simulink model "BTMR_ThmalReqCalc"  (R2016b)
settings: Solver=FixedStepDiscrete  StartTime=0.0  StopTime=10.0  FixedStep=0.1  RelTol=1e-3  EnableMultiTasking=on
undefined symbols (not defined in the file or in its folder): BMS_cntThmStbNum_C, BTMR_cntThmalReqVal_C, BTMR_flgCoolPwrCal_C, BTMR_pChrgClntPwrLv1_C, BTMR_pChrgClntPwrLv2_C, BTMR_pChrgClntPwrLv3_C, BTMR_pChrgClntPwrLv4_C, BTMR_pChrgClntPwrLv5_C, BTMR_pChrgClntPwrLv6_C, BTMR_pCoolPwrVal_C, BTMR_pHtgACPwrReq_C, BTMR_pHtgDCPwrReq_C, BTMR_pHtgDrvPwrReq_C, BTMR_pHtgsStage1_CUR, BTMR_pHtgsStage2_CUR, BTMR_pNormClntPwrLv1_C, BTMR_pNormClntPwrLv2_C, BTMR_pNormClntPwrLv3_C, BTMR_r861BrsDrvSoc_C, BTMR_r861HtgDrvSoc_C, BTMR_r891BrsDrvSoc_C, BTMR_r891HtgDrvSoc_C, BTMR_rCoolClbFlg_C, BTMR_rFlashClbFlg_C, BTMR_rHeatClbFlg_C, BTMR_t861BrsDiffLv0Temp_C, BTMR_t861BrsDiffLv1Temp_C, BTMR_t861CoolChrgAces2Temp_C, BTMR_t861CoolChrgAces3Temp_C, BTMR_t861CoolChrgAcesTemp_C, BTMR_t861CoolChrgDiffDebTemp_C, BTMR_t861CoolChrgEndDiffTemp_C, BTMR_t861CoolChrgExitLv2Temp_C, BTMR_t861CoolChrgExitLv3Temp_C, BTMR_t861CoolChrgExitTemp_C, BTMR_t861CoolChrgIntLv0Temp_C, BTMR_t861CoolChrgIntLv1Temp_C, BTMR_t861CoolChrgIntLv2Temp_C, BTMR_t861CoolChrgIntLv3Temp_C, BTMR_t861CoolChrgIntLv4Temp_C, BTMR_t861CoolChrgIntLv5Temp_C, BTMR_t861CoolDCDebTemp_C, BTMR_t861CoolNormAcesTemp_C, BTMR_t861CoolNormDiffDebTemp_C, BTMR_t861CoolNormEndDiffTemp_C, BTMR_t861CoolNormExitLv2Temp_C, BTMR_t861CoolNormExitLv3Temp_C, BTMR_t861CoolNormExitTemp_C, BTMR_t861CoolNormIntLv0Temp_C, BTMR_t861CoolNormIntLv1Temp_C, BTMR_t861CoolNormLv2Temp_C, BTMR_t861CoolNormLv3Temp_C, BTMR_t861HtgACDiffDebTemp_C, BTMR_t861HtgACEndDiffTemp_C, BTMR_t861HtgACStartHiTemp_C, BTMR_t861HtgACStartLoTemp_C, BTMR_t861HtgACStopTemp_C, BTMR_t861HtgDCDiffDebTemp_C, BTMR_t861HtgDCEndDiffTemp_C, BTMR_t861HtgDCIntLv0Temp_C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
libraries: AIWAYS_Powertrain_BMS_lib x78, simulink x9
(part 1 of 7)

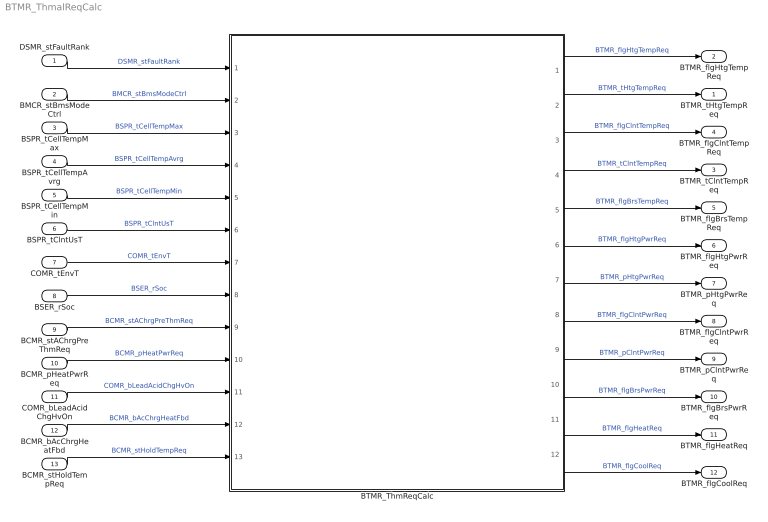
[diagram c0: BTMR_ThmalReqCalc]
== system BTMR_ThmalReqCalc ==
  DSMR_stFaultRank : Inport
  BMCR_stBmsModeCtrl : Inport  Port=2
  BSPR_tCellTempMax : Inport  Port=3
  BSPR_tCellTempAvrg : Inport  Port=4
  BSPR_tCellTempMin : Inport  Port=5
  BSPR_tClntUsT : Inport  Port=6
  COMR_tEnvT : Inport  Port=7
  BSER_rSoc : Inport  Port=8
  BCMR_stAChrgPreThmReq : Inport  Port=9
  BCMR_pHeatPwrReq : Inport  Port=10
  COMR_bLeadAcidChgHvOn : Inport  Port=11
  BCMR_bAcChrgHeatFbd : Inport  Port=12
  BCMR_stHoldTempReq : Inport  Port=13
  BTMR_ThmReqCalc : Subsystem
  BTMR_tHtgTempReq : Outport
  BTMR_flgHtgTempReq : Outport  Port=2
  BTMR_tClntTempReq : Outport  Port=3
  BTMR_flgClntTempReq : Outport  Port=4
  BTMR_flgBrsTempReq : Outport  Port=5
  BTMR_flgHtgPwrReq : Outport  Port=6
  BTMR_pHtgPwrReq : Outport  Port=7
  BTMR_flgClntPwrReq : Outport  Port=8
  BTMR_pClntPwrReq : Outport  Port=9
  BTMR_flgBrsPwrReq : Outport  Port=10
  BTMR_flgHeatReq : Outport  Port=11
  BTMR_flgCoolReq : Outport  Port=12
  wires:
  BMCR_stBmsModeCtrl/1 -> BTMR_ThmReqCalc/2(BMCR_stBmsModeCtrl)  "BMCR_stBmsModeCtrl"
  DSMR_stFaultRank/1 -> BTMR_ThmReqCalc/1(DSMR_stFaultRank)  "DSMR_stFaultRank"
  BSPR_tCellTempMax/1 -> BTMR_ThmReqCalc/3(BSPR_tCellTempMax)  "BSPR_tCellTempMax"
  BSPR_tCellTempAvrg/1 -> BTMR_ThmReqCalc/4(BSPR_tCellTempAvrg)  "BSPR_tCellTempAvrg"
  BSPR_tCellTempMin/1 -> BTMR_ThmReqCalc/5(BSPR_tCellTempMin)  "BSPR_tCellTempMin"
  BTMR_ThmReqCalc/2(BTMR_tHtgTempReq) -> BTMR_tHtgTempReq/1  "BTMR_tHtgTempReq"
  COMR_tEnvT/1 -> BTMR_ThmReqCalc/7(COMR_tEnvT)  "COMR_tEnvT"
  BSPR_tClntUsT/1 -> BTMR_ThmReqCalc/6(BSPR_tClntUsT)  "BSPR_tClntUsT"
  BSER_rSoc/1 -> BTMR_ThmReqCalc/8(BSER_rSoc)  "BSER_rSoc"
  BCMR_pHeatPwrReq/1 -> BTMR_ThmReqCalc/10(BCMR_pHeatPwrReq)  "BCMR_pHeatPwrReq"
  BCMR_stAChrgPreThmReq/1 -> BTMR_ThmReqCalc/9(BCMR_stAChrgPreThmReq)  "BCMR_stAChrgPreThmReq"
  BTMR_ThmReqCalc/1(BTMR_flgHtgTempReq) -> BTMR_flgHtgTempReq/1  "BTMR_flgHtgTempReq"
  BTMR_ThmReqCalc/5(BTMR_flgBrsTempReq) -> BTMR_flgBrsTempReq/1  "BTMR_flgBrsTempReq"
  BTMR_ThmReqCalc/4(BTMR_tClntTempReq) -> BTMR_tClntTempReq/1  "BTMR_tClntTempReq"
  BTMR_ThmReqCalc/3(BTMR_flgClntTempReq) -> BTMR_flgClntTempReq/1  "BTMR_flgClntTempReq"
  COMR_bLeadAcidChgHvOn/1 -> BTMR_ThmReqCalc/11(COMR_bLeadAcidChgHvOn)  "COMR_bLeadAcidChgHvOn"
  BCMR_bAcChrgHeatFbd/1 -> BTMR_ThmReqCalc/12(BCMR_bAcChrgHeatFbd)  "BCMR_bAcChrgHeatFbd"
  BTMR_ThmReqCalc/6(BTMR_flgHtgPwrReq) -> BTMR_flgHtgPwrReq/1  "BTMR_flgHtgPwrReq"
  BTMR_ThmReqCalc/7(BTMR_pHtgPwrReq) -> BTMR_pHtgPwrReq/1  "BTMR_pHtgPwrReq"
  BTMR_ThmReqCalc/8(BTMR_flgClntPwrReq) -> BTMR_flgClntPwrReq/1  "BTMR_flgClntPwrReq"
  BTMR_ThmReqCalc/9(BTMR_pClntPwrReq) -> BTMR_pClntPwrReq/1  "BTMR_pClntPwrReq"
  BTMR_ThmReqCalc/10(BTMR_flgBrsPwrReq) -> BTMR_flgBrsPwrReq/1  "BTMR_flgBrsPwrReq"
  BCMR_stHoldTempReq/1 -> BTMR_ThmReqCalc/13(BCMR_stHoldTempReq)  "BCMR_stHoldTempReq"
  BTMR_ThmReqCalc/11(BTMR_flgHeatReq) -> BTMR_flgHeatReq/1  "BTMR_flgHeatReq"
  BTMR_ThmReqCalc/12(BTMR_flgCoolReq) -> BTMR_flgCoolReq/1  "BTMR_flgCoolReq"

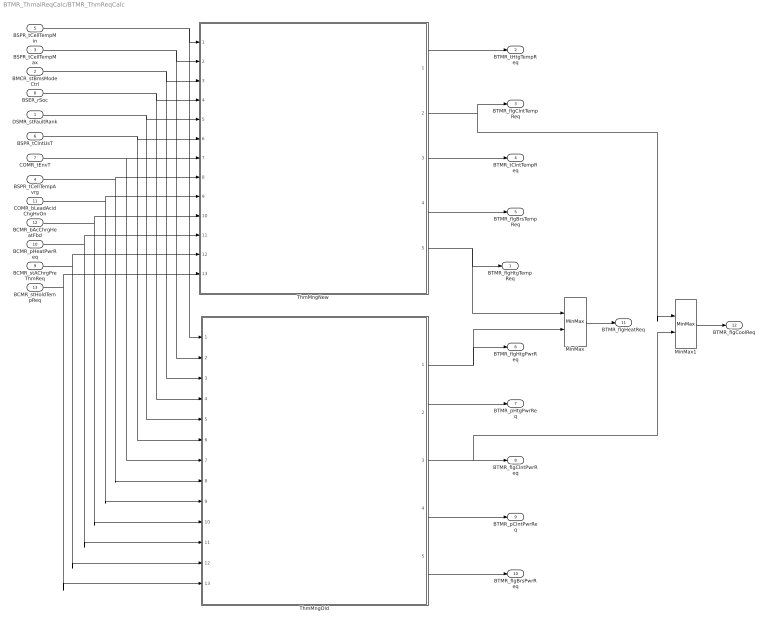
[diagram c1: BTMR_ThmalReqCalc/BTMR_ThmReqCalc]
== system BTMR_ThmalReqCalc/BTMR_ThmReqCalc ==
  DSMR_stFaultRank : Inport
  BMCR_stBmsModeCtrl : Inport  Port=2
  BSPR_tCellTempMax : Inport  Port=3
  BSPR_tCellTempAvrg : Inport  Port=4
  BSPR_tCellTempMin : Inport  Port=5
  BSPR_tClntUsT : Inport  Port=6
  COMR_tEnvT : Inport  Port=7
  BSER_rSoc : Inport  Port=8
  BCMR_stAChrgPreThmReq : Inport  Port=9
  BCMR_pHeatPwrReq : Inport  Port=10
  COMR_bLeadAcidChgHvOn : Inport  Port=11
  BCMR_bAcChrgHeatFbd : Inport  Port=12
  BCMR_stHoldTempReq : Inport  Port=13
  MinMax : MinMax  Function=max  Inputs=2
  MinMax1 : MinMax  Function=max  Inputs=2
  ThmMngNew : Subsystem
  ThmMngOld : Subsystem
  BTMR_flgHtgTempReq : Outport
  BTMR_tHtgTempReq : Outport  Port=2
  BTMR_flgClntTempReq : Outport  Port=3
  BTMR_tClntTempReq : Outport  Port=4
  BTMR_flgBrsTempReq : Outport  Port=5
  BTMR_flgHtgPwrReq : Outport  Port=6
  BTMR_pHtgPwrReq : Outport  Port=7
  BTMR_flgClntPwrReq : Outport  Port=8
  BTMR_pClntPwrReq : Outport  Port=9
  BTMR_flgBrsPwrReq : Outport  Port=10
  BTMR_flgHeatReq : Outport  Port=11
  BTMR_flgCoolReq : Outport  Port=12
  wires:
  BSPR_tCellTempMin/1 -> ThmMngOld/1(BSPR_tCellTempMin), ThmMngNew/1(BSPR_tCellTempMin)
  BSPR_tCellTempMax/1 -> ThmMngOld/2(BSPR_tCellTempMax), ThmMngNew/2(BSPR_tCellTempMax)
  BMCR_stBmsModeCtrl/1 -> ThmMngOld/3(BMCR_stBmsModeCtrl), ThmMngNew/3(BMCR_stBmsModeCtrl)
  BSER_rSoc/1 -> ThmMngOld/4(BSER_rSoc), ThmMngNew/4(BSER_rSoc)
  DSMR_stFaultRank/1 -> ThmMngOld/5(DSMR_stFaultRank), ThmMngNew/5(DSMR_stFaultRank)
  BSPR_tClntUsT/1 -> ThmMngOld/6(BSPR_tClntUsT), ThmMngNew/6(BSPR_tClntUsT)
  COMR_tEnvT/1 -> ThmMngOld/7(COMR_tEnvT), ThmMngNew/7(COMR_tEnvT)
  BSPR_tCellTempAvrg/1 -> ThmMngOld/8(BSPR_tCellTempAvrg), ThmMngNew/8(BSPR_tCellTempAvrg)
  COMR_bLeadAcidChgHvOn/1 -> ThmMngOld/9(COMR_bLeadAcidChgHvOn), ThmMngNew/9(COMR_bLeadAcidChgHvOn)
  BCMR_bAcChrgHeatFbd/1 -> ThmMngOld/10(BCMR_bAcChrgHeatFbd), ThmMngNew/10(BCMR_bAcChrgHeatFbd)
  BCMR_pHeatPwrReq/1 -> ThmMngOld/11(BCMR_pHeatPwrReq), ThmMngNew/11(BCMR_pHeatPwrReq)
  BCMR_stAChrgPreThmReq/1 -> ThmMngOld/12(BCMR_stAChrgPreThmReq), ThmMngNew/12(BCMR_stAChrgPreThmReq)
  ThmMngNew/5(BTMR_flgHtgTempReq_891) -> MinMax/1, BTMR_flgHtgTempReq/1
  ThmMngNew/1(BTMR_tHtgTempReq_891) -> BTMR_tHtgTempReq/1
  ThmMngNew/2(BTMR_flgClntTempReq_891) -> MinMax1/1, BTMR_flgClntTempReq/1
  ThmMngNew/3(BTMR_tClntTempReq_891) -> BTMR_tClntTempReq/1
  ThmMngNew/4(BTMR_flgBrsTempReq_891) -> BTMR_flgBrsTempReq/1
  ThmMngOld/1(BTMR_flgHtgPwrReq_861) -> BTMR_flgHtgPwrReq/1, MinMax/2
  ThmMngOld/2(BTMR_pHtgPwrReq_861) -> BTMR_pHtgPwrReq/1
  ThmMngOld/3(BTMR_flgClntPwrReq_861) -> MinMax1/2, BTMR_flgClntPwrReq/1
  ThmMngOld/4(BTMR_pClntPwrReq_861) -> BTMR_pClntPwrReq/1
  ThmMngOld/5(BTMR_flgBrsPwrReq_861) -> BTMR_flgBrsPwrReq/1
  BCMR_stHoldTempReq/1 -> ThmMngNew/13(BCMR_stHoldTempReq), ThmMngOld/13(BCMR_stHoldTempReq)
  MinMax/1 -> BTMR_flgHeatReq/1
  MinMax1/1 -> BTMR_flgCoolReq/1

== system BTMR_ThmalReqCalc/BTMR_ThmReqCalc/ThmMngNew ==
  BSPR_tCellTempMin : Inport
  BSPR_tCellTempMax : Inport  Port=2
  BMCR_stBmsModeCtrl : Inport  Port=3
  BSER_rSoc : Inport  Port=4
  DSMR_stFaultRank : Inport  Port=5
  BSPR_tClntUsT : Inport  Port=6
  COMR_tEnvT : Inport  Port=7
  BSPR_tCellTempAvrg : Inport  Port=8
  COMR_bLeadAcidChgHvOn : Inport  Port=9
  BCMR_bAcChrgHeatFbd : Inport  Port=10
  BCMR_pHeatPwrReq : Inport  Port=11
  BCMR_stAChrgPreThmReq : Inport  Port=12
  BCMR_stHoldTempReq : Inport  Port=13
  BTMR_ThmFlgTempCalc : Subsystem
  BTMR_ThmLogSgnsCalc : Subsystem
  BTMR_ThmSgnsPros : Subsystem
  BTMR_ThmStsCalc : Subsystem
  BTMR_tHtgTempReq_891 : Outport
  BTMR_flgClntTempReq_891 : Outport  Port=2
  BTMR_tClntTempReq_891 : Outport  Port=3
  BTMR_flgBrsTempReq_891 : Outport  Port=4
  BTMR_flgHtgTempReq_891 : Outport  Port=5
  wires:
  COMR_tEnvT/1 -> BTMR_ThmSgnsPros/7(COMR_tEnvT)
  BTMR_ThmStsCalc/1(stBrsSts) -> BTMR_ThmFlgTempCalc/1(stBrsSts)
  BTMR_ThmStsCalc/2(stHtgSts) -> BTMR_ThmFlgTempCalc/2(stHtgSts)
  BTMR_ThmStsCalc/3(stCoolSts) -> BTMR_ThmFlgTempCalc/3(stCoolSts)
  BTMR_ThmFlgTempCalc/5(BTMR_flgBrsTempReq) -> BTMR_flgBrsTempReq_891/1
  BTMR_ThmFlgTempCalc/1(BTMR_flgHtgTempReq) -> BTMR_flgHtgTempReq_891/1
  BTMR_ThmFlgTempCalc/2(BTMR_tHtgTempReq) -> BTMR_tHtgTempReq_891/1
  BTMR_ThmFlgTempCalc/3(BTMR_flgClntTempReq) -> BTMR_flgClntTempReq_891/1
  BTMR_ThmFlgTempCalc/4(BTMR_tClntTempReq) -> BTMR_tClntTempReq_891/1
  BSPR_tCellTempMin/1 -> BTMR_ThmSgnsPros/1(BSPR_tCellTempMin)
  BSPR_tCellTempMax/1 -> BTMR_ThmSgnsPros/2(BSPR_tCellTempMax)
  BSER_rSoc/1 -> BTMR_ThmSgnsPros/4(BSER_rSoc)
  BMCR_stBmsModeCtrl/1 -> BTMR_ThmSgnsPros/3(BMCR_stBmsModeCtrl)
  DSMR_stFaultRank/1 -> BTMR_ThmSgnsPros/5(DSMR_stFaultRank)
  BSPR_tClntUsT/1 -> BTMR_ThmSgnsPros/6(BSPR_tClntUsT)
  BTMR_ThmSgnsPros/3(BTMR_flgThmEnaTempSgns) -> BTMR_ThmLogSgnsCalc/3(BTMR_flgThmEnaTempSgns)
  BTMR_ThmSgnsPros/4(BTMR_flgBrsTempSgns) -> BTMR_ThmStsCalc/4(BTMR_flgBrsTempSgns), BTMR_ThmLogSgnsCalc/4(BTMR_flgBrsTempSgns)
  BTMR_ThmSgnsPros/1(BTMR_flgBMSStsSgns) -> BTMR_ThmLogSgnsCalc/1(BTMR_flgBMSStsSgns)
  BTMR_ThmSgnsPros/2(BTMR_flgSOCSgns) -> BTMR_ThmLogSgnsCalc/2(BTMR_flgSOCSgns)
  BTMR_ThmSgnsPros/6(BTMR_flgCoolTempSgns) -> BTMR_ThmLogSgnsCalc/6(BTMR_flgCoolTempSgns), BTMR_ThmFlgTempCalc/4(BTMR_flgCoolTempSgns)
  BTMR_ThmSgnsPros/5(BTMR_flgHtgTempSgns) -> BTMR_ThmLogSgnsCalc/5(BTMR_flgHtgTempSgns)
  BTMR_ThmLogSgnsCalc/1(BTMR_flgBTMREnaSgns) -> BTMR_ThmStsCalc/1(BTMR_flgBTMREnaSgns)
  BTMR_ThmLogSgnsCalc/2(BTMR_flgBTMRDnaSgns) -> BTMR_ThmStsCalc/2(BTMR_flgBTMRDnaSgns)
  BTMR_ThmSgnsPros/7(BTMR_flgThmEndSgns) -> BTMR_ThmStsCalc/3(BTMR_flgThmEndSgns)
  BSPR_tCellTempAvrg/1 -> BTMR_ThmSgnsPros/8(BSPR_tCellTempAvrg)
  COMR_bLeadAcidChgHvOn/1 -> BTMR_ThmSgnsPros/9(COMR_bLeadAcidChgHvOn)
  BCMR_pHeatPwrReq/1 -> BTMR_ThmFlgTempCalc/5(BCMR_pHeatPwrReq)
  BCMR_stAChrgPreThmReq/1 -> BTMR_ThmFlgTempCalc/6(BCMR_stAChrgPreThmReq)
  BCMR_bAcChrgHeatFbd/1 -> BTMR_ThmSgnsPros/10(BCMR_bAcChrgHeatFbd)
  BCMR_stHoldTempReq/1 -> BTMR_ThmFlgTempCalc/7(BCMR_stHoldTempReq)

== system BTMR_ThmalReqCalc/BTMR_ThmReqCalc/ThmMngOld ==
  BSPR_tCellTempMin : Inport
  BSPR_tCellTempMax : Inport  Port=2
  BMCR_stBmsModeCtrl : Inport  Port=3
  BSER_rSoc : Inport  Port=4
  DSMR_stFaultRank : Inport  Port=5
  BSPR_tClntUsT : Inport  Port=6
  COMR_tEnvT : Inport  Port=7
  BSPR_tCellTempAvrg : Inport  Port=8
  COMR_bLeadAcidChgHvOn : Inport  Port=9
  BCMR_bAcChrgHeatFbd : Inport  Port=10
  BCMR_pHeatPwrReq : Inport  Port=11
  BCMR_stAChrgPreThmReq : Inport  Port=12
  BCMR_stHoldTempReq : Inport  Port=13
  BTMR_ThmFlgPwrCalc : Subsystem
  BTMR_ThmInSgnsPros : Subsystem
  BTMR_ThmLogSgnsCalc : Subsystem
  BTMR_ThmStsCalc : Subsystem
  BTMR_flgHtgPwrReq_861 : Outport
  BTMR_pHtgPwrReq_861 : Outport  Port=2
  BTMR_flgClntPwrReq_861 : Outport  Port=3
  BTMR_pClntPwrReq_861 : Outport  Port=4
  BTMR_flgBrsPwrReq_861 : Outport  Port=5
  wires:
  COMR_tEnvT/1 -> BTMR_ThmInSgnsPros/7(COMR_tEnvT)
  BTMR_ThmStsCalc/1(stBrsSts) -> BTMR_ThmFlgPwrCalc/1(stBrsSts)
  BTMR_ThmStsCalc/2(stHtgSts) -> BTMR_ThmFlgPwrCalc/2(stHtgSts)
  BTMR_ThmStsCalc/3(stCoolSts) -> BTMR_ThmFlgPwrCalc/3(stCoolSts)
  BTMR_ThmFlgPwrCalc/5(BTMR_flgBrsPwrReq) -> BTMR_flgBrsPwrReq_861/1
  BTMR_ThmFlgPwrCalc/1(BTMR_flgHtgPwrReq) -> BTMR_flgHtgPwrReq_861/1
  BTMR_ThmFlgPwrCalc/2(BTMR_pHtgPwrReq) -> BTMR_pHtgPwrReq_861/1
  BTMR_ThmFlgPwrCalc/3(BTMR_flgClntPwrReq) -> BTMR_flgClntPwrReq_861/1
  BTMR_ThmFlgPwrCalc/4(BTMR_pClntPwrReq) -> BTMR_pClntPwrReq_861/1
  BSPR_tCellTempMin/1 -> BTMR_ThmInSgnsPros/1(BSPR_tCellTempMin)
  BSPR_tCellTempMax/1 -> BTMR_ThmInSgnsPros/2(BSPR_tCellTempMax)
  BSER_rSoc/1 -> BTMR_ThmInSgnsPros/4(BSER_rSoc)
  BMCR_stBmsModeCtrl/1 -> BTMR_ThmInSgnsPros/3(BMCR_stBmsModeCtrl)
  DSMR_stFaultRank/1 -> BTMR_ThmInSgnsPros/5(DSMR_stFaultRank)
  BSPR_tClntUsT/1 -> BTMR_ThmInSgnsPros/6(BSPR_tClntUsT)
  BTMR_ThmInSgnsPros/3(BTMR_flgThmEnaTempSgns) -> BTMR_ThmLogSgnsCalc/3(BTMR_flgThmEnaTempSgns)
  BTMR_ThmInSgnsPros/4(BTMR_flgBrsTempSgns) -> BTMR_ThmLogSgnsCalc/4(BTMR_flgBrsTempSgns), BTMR_ThmStsCalc/4(BTMR_flgBrsTempSgns)
  BTMR_ThmInSgnsPros/1(BTMR_flgBMSStsSgns) -> BTMR_ThmLogSgnsCalc/1(BTMR_flgBMSStsSgns)
  BTMR_ThmInSgnsPros/2(BTMR_flgSOCSgns) -> BTMR_ThmLogSgnsCalc/2(BTMR_flgSOCSgns)
  BTMR_ThmInSgnsPros/6(BTMR_flgCoolTempSgns) -> BTMR_ThmLogSgnsCalc/6(BTMR_flgCoolTempSgns), BTMR_ThmFlgPwrCalc/5(BTMR_flgCoolTempSgns)
  BTMR_ThmInSgnsPros/5(BTMR_flgHtgTempSgns) -> BTMR_ThmLogSgnsCalc/5(BTMR_flgHtgTempSgns), BTMR_ThmFlgPwrCalc/4(BTMR_flgHtgTempSgns)
  BTMR_ThmLogSgnsCalc/1(BTMR_flgBTMREnaSgns) -> BTMR_ThmStsCalc/1(BTMR_flgBTMREnaSgns)
  BTMR_ThmLogSgnsCalc/2(BTMR_flgBTMRDnaSgns) -> BTMR_ThmStsCalc/2(BTMR_flgBTMRDnaSgns)
  BTMR_ThmInSgnsPros/7(BTMR_flgThmEndSgns) -> BTMR_ThmStsCalc/3(BTMR_flgThmEndSgns)
  BTMR_ThmInSgnsPros/8(BTMR_pHtgDCPwrSgns) -> BTMR_ThmFlgPwrCalc/6(BTMR_pHtgDCPwrSgns)
  BSPR_tCellTempAvrg/1 -> BTMR_ThmInSgnsPros/8(BSPR_tCellTempAvrg)
  COMR_bLeadAcidChgHvOn/1 -> BTMR_ThmInSgnsPros/9(COMR_bLeadAcidChgHvOn)
  BCMR_pHeatPwrReq/1 -> BTMR_ThmFlgPwrCalc/7(BCMR_pHeatPwrReq)
  BCMR_stAChrgPreThmReq/1 -> BTMR_ThmFlgPwrCalc/8(BCMR_stAChrgPreThmReq)
  BCMR_bAcChrgHeatFbd/1 -> BTMR_ThmInSgnsPros/10(BCMR_bAcChrgHeatFbd)
  BCMR_stHoldTempReq/1 -> BTMR_ThmFlgPwrCalc/9(BCMR_stHoldTempReq)

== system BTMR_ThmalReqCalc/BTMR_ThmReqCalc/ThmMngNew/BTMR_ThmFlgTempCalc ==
  stBrsSts : Inport
  stHtgSts : Inport  Port=2
  stCoolSts : Inport  Port=3
  BTMR_flgCoolTempSgns : Inport  Port=4
  BCMR_pHeatPwrReq : Inport  Port=5
  BCMR_stAChrgPreThmReq : Inport  Port=6
  BCMR_stHoldTempReq : Inport  Port=7
  BTMR_BrushFlgCalc : Subsystem  TreatAsAtomicUnit=on
  BTMR_CoolFlgTempCalc : Subsystem
  BTMR_HtgFlgTempCalc : Subsystem  TreatAsAtomicUnit=on
  BTMR_flgHtgTempReq : Outport
  BTMR_tHtgTempReq : Outport  Port=2
  BTMR_flgClntTempReq : Outport  Port=3
  BTMR_tClntTempReq : Outport  Port=4
  BTMR_flgBrsTempReq : Outport  Port=5
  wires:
  BTMR_CoolFlgTempCalc/1(BTMR_flgClntTempReq) -> BTMR_flgClntTempReq/1
  BTMR_CoolFlgTempCalc/2(BTMR_tClntTempReq) -> BTMR_tClntTempReq/1
  BTMR_BrushFlgCalc/1(BTMR_flgBrsTempReq) -> BTMR_CoolFlgTempCalc/1(BTMR_flgBrsTempReq), BTMR_flgBrsTempReq/1
  BTMR_HtgFlgTempCalc/1(BTMR_flgHtgTempReq) -> BTMR_flgHtgTempReq/1
  BTMR_HtgFlgTempCalc/2(BTMR_tHtgTempReq) -> BTMR_tHtgTempReq/1
  stBrsSts/1 -> BTMR_BrushFlgCalc/1(stBrsSts)
  stHtgSts/1 -> BTMR_HtgFlgTempCalc/1(stHtgSts)
  stCoolSts/1 -> BTMR_CoolFlgTempCalc/2(stCoolSts)
  BTMR_flgCoolTempSgns/1 -> BTMR_CoolFlgTempCalc/3(BTMR_flgCoolTempSgns)
  BCMR_pHeatPwrReq/1 -> BTMR_HtgFlgTempCalc/2(BCMR_pHeatPwrReq)
  BCMR_stAChrgPreThmReq/1 -> BTMR_HtgFlgTempCalc/3(BCMR_stAChrgPreThmReq)
  BCMR_stHoldTempReq/1 -> BTMR_HtgFlgTempCalc/4(BCMR_stHoldTempReq)

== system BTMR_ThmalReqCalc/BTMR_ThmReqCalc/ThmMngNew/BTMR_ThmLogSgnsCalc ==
  BTMR_flgBMSStsSgns : Inport
  BTMR_flgSOCSgns : Inport  Port=2
  BTMR_flgThmEnaTempSgns : Inport  Port=3
  BTMR_flgBrsTempSgns : Inport  Port=4
  BTMR_flgHtgTempSgns : Inport  Port=5
  BTMR_flgCoolTempSgns : Inport  Port=6
  BTMR_BThmDnaLogCalc : Subsystem
  BTMR_BThmEnaLogCalc : Subsystem
  BTMR_ThmLogPreCalc : Subsystem
  BTMR_flgBTMREnaSgns : Outport
  BTMR_flgBTMRDnaSgns : Outport  Port=2
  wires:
  BTMR_flgBrsTempSgns/1 -> BTMR_BThmDnaLogCalc/2(BTMR_flgBrsTempSgns), BTMR_ThmLogPreCalc/4(BTMR_flgBrsTempSgns)
  BTMR_flgHtgTempSgns/1 -> BTMR_BThmDnaLogCalc/3(BTMR_flgHtgTempSgns)
  BTMR_flgCoolTempSgns/1 -> BTMR_BThmDnaLogCalc/4(BTMR_flgCoolTempSgns)
  BTMR_BThmDnaLogCalc/1(BTMR_flgBThmDnaSgns) -> BTMR_flgBTMRDnaSgns/1
  BTMR_flgBMSStsSgns/1 -> BTMR_ThmLogPreCalc/1(BTMR_flgBMSStsSgns)
  BTMR_flgSOCSgns/1 -> BTMR_BThmEnaLogCalc/4(BTMR_flgSOCSgns), BTMR_BThmDnaLogCalc/1(BTMR_flgSOCSgns), BTMR_ThmLogPreCalc/2(BTMR_flgSOCSgns)
  BTMR_BThmEnaLogCalc/1(BTMR_flgBTMREnaSgns) -> BTMR_flgBTMREnaSgns/1
  BTMR_ThmLogPreCalc/2(BTMR_flgHtgLogSgns) -> BTMR_BThmEnaLogCalc/2(BTMR_flgHtgLogSgns)
  BTMR_ThmLogPreCalc/1(BTMR_flgBrsLogSgns) -> BTMR_BThmEnaLogCalc/1(BTMR_flgBrsLogSgns)
  BTMR_ThmLogPreCalc/3(BTMR_flgCoolLogSgns) -> BTMR_BThmEnaLogCalc/3(BTMR_flgCoolLogSgns)
  BTMR_flgThmEnaTempSgns/1 -> BTMR_ThmLogPreCalc/3(BTMR_flgThmEnaTempSgns)

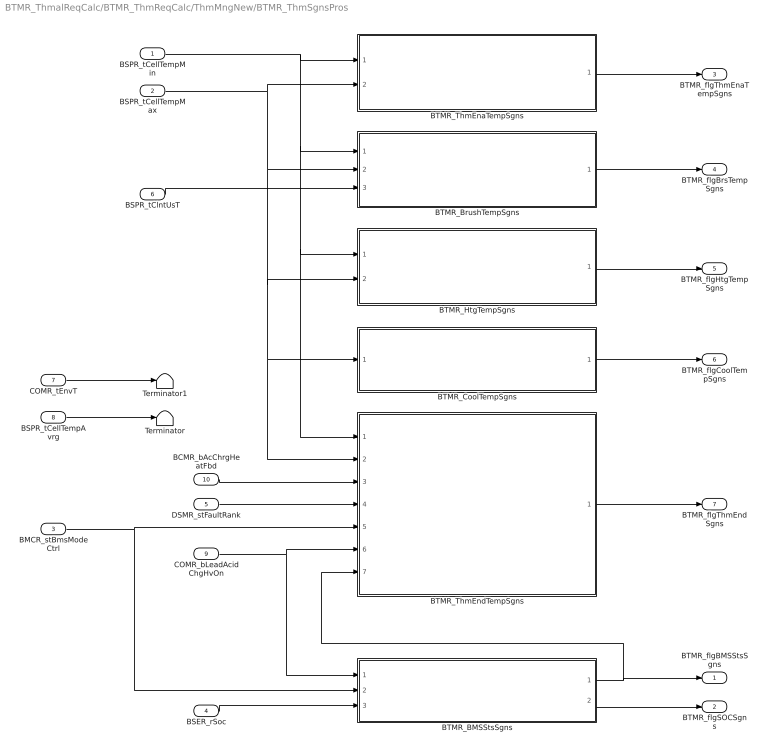
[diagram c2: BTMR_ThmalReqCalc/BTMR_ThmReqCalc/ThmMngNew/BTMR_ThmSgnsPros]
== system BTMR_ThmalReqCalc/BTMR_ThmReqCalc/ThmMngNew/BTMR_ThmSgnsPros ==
  BSPR_tCellTempMin : Inport
  BSPR_tCellTempMax : Inport  Port=2
  BMCR_stBmsModeCtrl : Inport  Port=3
  BSER_rSoc : Inport  Port=4
  DSMR_stFaultRank : Inport  Port=5
  BSPR_tClntUsT : Inport  Port=6
  COMR_tEnvT : Inport  Port=7
  BSPR_tCellTempAvrg : Inport  Port=8
  COMR_bLeadAcidChgHvOn : Inport  Port=9
  BCMR_bAcChrgHeatFbd : Inport  Port=10
  BTMR_BMSStsSgns : Subsystem
  BTMR_BrushTempSgns : Subsystem
  BTMR_CoolTempSgns : Subsystem
  BTMR_HtgTempSgns : Subsystem
  BTMR_ThmEnaTempSgns : Subsystem
  BTMR_ThmEndTempSgns : Subsystem
  Terminator : Terminator
  Terminator1 : Terminator
  BTMR_flgBMSStsSgns : Outport
  BTMR_flgSOCSgns : Outport  Port=2
  BTMR_flgThmEnaTempSgns : Outport  Port=3
  BTMR_flgBrsTempSgns : Outport  Port=4
  BTMR_flgHtgTempSgns : Outport  Port=5
  BTMR_flgCoolTempSgns : Outport  Port=6
  BTMR_flgThmEndSgns : Outport  Port=7
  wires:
  BTMR_ThmEnaTempSgns/1(BTMR_flgThmEnaTempSgns) -> BTMR_flgThmEnaTempSgns/1
  BSPR_tClntUsT/1 -> BTMR_BrushTempSgns/3(BSPR_tClntUsT)
  BTMR_CoolTempSgns/1(BTMR_flgCoolTempSgns) -> BTMR_flgCoolTempSgns/1
  BSER_rSoc/1 -> BTMR_BMSStsSgns/3(BSER_rSoc)
  BTMR_ThmEndTempSgns/1(BTMR_flgThmEndSgns) -> BTMR_flgThmEndSgns/1
  BTMR_BMSStsSgns/1(BTMR_flgBMSSgns) -> BTMR_ThmEndTempSgns/7(BTMR_flgBMSSgns), BTMR_flgBMSStsSgns/1
  BTMR_HtgTempSgns/1(BTMR_flgHtgTempSgns) -> BTMR_flgHtgTempSgns/1
  BTMR_BrushTempSgns/1(BTMR_flgBrsTempSgns) -> BTMR_flgBrsTempSgns/1
  BTMR_BMSStsSgns/2(BTMR_flgSOCSgns) -> BTMR_flgSOCSgns/1
  BMCR_stBmsModeCtrl/1 -> BTMR_BMSStsSgns/2(BMCR_stBmsModeCtrl), BTMR_ThmEndTempSgns/5(BMCR_stBmsModeCtrl)
  DSMR_stFaultRank/1 -> BTMR_ThmEndTempSgns/4(DSMR_stFaultRank)
  BSPR_tCellTempMax/1 -> BTMR_ThmEndTempSgns/2(BSPR_tCellTempMax), BTMR_CoolTempSgns/1(BSPR_tCellTempMax), BTMR_HtgTempSgns/2(BSPR_tCellTempMax), BTMR_BrushTempSgns/2(BSPR_tCellTempMax), BTMR_ThmEnaTempSgns/2(BSPR_tCellTempMax)
  BSPR_tCellTempMin/1 -> BTMR_ThmEndTempSgns/1(BSPR_tCellTempMin), BTMR_HtgTempSgns/1(BSPR_tCellTempMin), BTMR_BrushTempSgns/1(BSPR_tCellTempMin), BTMR_ThmEnaTempSgns/1(BSPR_tCellTempMin)
  BSPR_tCellTempAvrg/1 -> Terminator/1
  COMR_bLeadAcidChgHvOn/1 -> BTMR_BMSStsSgns/1(COMR_bLeadAcidChgHvOn), BTMR_ThmEndTempSgns/6(COMR_bLeadAcidChgHvOn)
  COMR_tEnvT/1 -> Terminator1/1
  BCMR_bAcChrgHeatFbd/1 -> BTMR_ThmEndTempSgns/3(BCMR_bAcChrgHeatFbd)

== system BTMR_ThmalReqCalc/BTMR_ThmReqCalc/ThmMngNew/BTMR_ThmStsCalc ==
  BTMR_flgBTMREnaSgns : Inport
  BTMR_flgBTMRDnaSgns : Inport  Port=2
  BTMR_flgThmEndSgns : Inport  Port=3
  BTMR_flgBrsTempSgns : Inport  Port=4
  BTMR_ThmStsCalc : Stateflow chart  TreatAsAtomicUnit=on
  Bus Selector : BusSelector  OutputSignals=BTMR_flgBrsEna,BTMR_flgHtgDCEna,BTMR_flgHtgACEna,BTMR_flgHtgDrvSEna,BTMR_flgCoolNormEna,BTMR_flgCoolChrgEna
  Bus Selector1 : BusSelector  OutputSignals=BTMR_flgBrsDna,BTMR_flgHtgDCDna,BTMR_flgHtgACDna,BTMR_flgHtgDrvDna,BTMR_flgCoolNormDna,BTMR_flgCoolChrgDna
  Bus Selector2 : BusSelector  OutputSignals=BTMR_flgBrsThmEnd,BTMR_flgHtgDCThmEnd,BTMR_flgHtgACThmEnd,BTMR_flgHtgDrvThmEnd,BTMR_flgCoolNormThmEnd,BTMR_flgCoolChrgThmEnd
  Bus Selector3 : BusSelector  OutputSignals=BTMR_flgBrsInTempSgns
  Bus Selector4 : BusSelector  OutputSignals=BTMR_flgBrsStartTemp
  Data Type Conversion : DataTypeConversion  OutDataTypeStr=uint8
  Data Type Conversion1 : DataTypeConversion  OutDataTypeStr=uint8
  Data Type Conversion2 : DataTypeConversion  OutDataTypeStr=uint8
  stBrsSts : Outport
  stHtgSts : Outport  Port=2
  stCoolSts : Outport  Port=3
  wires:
  BTMR_ThmStsCalc/2(stHtgSts) -> Data Type Conversion1/1
  BTMR_ThmStsCalc/1(stBrsSts) -> Data Type Conversion/1
  BTMR_ThmStsCalc/3(stCoolSts) -> Data Type Conversion2/1
  BTMR_flgBTMREnaSgns/1 -> Bus Selector/1
  Bus Selector/2 -> BTMR_ThmStsCalc/2(HtgDCEna)  "<BTMR_flgHtgDCEna>"
  Bus Selector/1 -> BTMR_ThmStsCalc/1(BrsEna)  "<BTMR_flgBrsEna>"
  Bus Selector/3 -> BTMR_ThmStsCalc/3(HtgACEna)  "<BTMR_flgHtgACEna>"
  Bus Selector/4 -> BTMR_ThmStsCalc/4(HtgDrvEna)  "<BTMR_flgHtgDrvSEna>"
  Bus Selector/5 -> BTMR_ThmStsCalc/5(CoolNormEna)  "<BTMR_flgCoolNormEna>"
  Bus Selector/6 -> BTMR_ThmStsCalc/6(CoolChrgEna)  "<BTMR_flgCoolChrgEna>"
  BTMR_flgBTMRDnaSgns/1 -> Bus Selector1/1
  Bus Selector1/1 -> BTMR_ThmStsCalc/7(BrsDna)  "<BTMR_flgBrsDna>"
  Bus Selector1/2 -> BTMR_ThmStsCalc/8(HtgDCDna)  "<BTMR_flgHtgDCDna>"
  Bus Selector1/3 -> BTMR_ThmStsCalc/9(HtgACDna)  "<BTMR_flgHtgACDna>"
  Bus Selector1/4 -> BTMR_ThmStsCalc/10(HtgDrvDna)  "<BTMR_flgHtgDrvDna>"
  Bus Selector1/5 -> BTMR_ThmStsCalc/11(CoolNormDna)  "<BTMR_flgCoolNormDna>"
  Bus Selector1/6 -> BTMR_ThmStsCalc/12(CoolChrgDna)  "<BTMR_flgCoolChrgDna>"
  BTMR_flgThmEndSgns/1 -> Bus Selector2/1
  Bus Selector2/2 -> BTMR_ThmStsCalc/14(HtgDCThmEnd)  "<BTMR_flgHtgDCThmEnd>"
  Bus Selector2/3 -> BTMR_ThmStsCalc/15(HtgACThmEnd)  "<BTMR_flgHtgACThmEnd>"
  Bus Selector2/4 -> BTMR_ThmStsCalc/16(HtgDrvThmEnd)  "<BTMR_flgHtgDrvThmEnd>"
  Bus Selector2/5 -> BTMR_ThmStsCalc/17(CoolNormThmEnd)  "<BTMR_flgCoolNormThmEnd>"
  Bus Selector2/6 -> BTMR_ThmStsCalc/18(CoolChrgThmEnd)  "<BTMR_flgCoolChrgThmEnd>"
  BTMR_flgBrsTempSgns/1 -> Bus Selector3/1
  Bus Selector3/1 -> Bus Selector4/1  "<BTMR_flgBrsInTempSgns>"
  Bus Selector4/1 -> BTMR_ThmStsCalc/19(BrsStart)  "<BTMR_flgBrsStartTemp>"
  Bus Selector2/1 -> BTMR_ThmStsCalc/13(BrsThmEnd)  "<BTMR_flgBrsThmEnd>"
  Data Type Conversion/1 -> stBrsSts/1
  Data Type Conversion1/1 -> stHtgSts/1
  Data Type Conversion2/1 -> stCoolSts/1

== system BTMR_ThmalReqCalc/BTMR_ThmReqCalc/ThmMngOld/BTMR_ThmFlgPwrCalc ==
  stBrsSts : Inport
  stHtgSts : Inport  Port=2
  stCoolSts : Inport  Port=3
  BTMR_flgHtgTempSgns : Inport  Port=4
  BTMR_flgCoolTempSgns : Inport  Port=5
  BTMR_pHtgDCPwrSgns : Inport  Port=6
  BCMR_pHeatPwrReq : Inport  Port=7
  BCMR_stAChrgPreThmReq : Inport  Port=8
  BCMR_stHoldTempReq : Inport  Port=9
  BTMR_BrushFlgCalc : Subsystem  TreatAsAtomicUnit=on
  BTMR_CoolFlgPwrCalc : Subsystem
  BTMR_HtgFlgPwrCalc : Subsystem  TreatAsAtomicUnit=on
  BTMR_flgHtgPwrReq : Outport
  BTMR_pHtgPwrReq : Outport  Port=2
  BTMR_flgClntPwrReq : Outport  Port=3
  BTMR_pClntPwrReq : Outport  Port=4
  BTMR_flgBrsPwrReq : Outport  Port=5
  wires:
  BTMR_CoolFlgPwrCalc/1(BTMR_flgClntPwrReq) -> BTMR_flgClntPwrReq/1
  BTMR_CoolFlgPwrCalc/2(BTMR_pClntPwrReq) -> BTMR_pClntPwrReq/1
  BTMR_BrushFlgCalc/1(BTMR_flgBrsPwrReq) -> BTMR_CoolFlgPwrCalc/1(BTMR_flgBrsPwrReq), BTMR_flgBrsPwrReq/1
  BTMR_HtgFlgPwrCalc/1(BTMR_flgHtgPwrReq) -> BTMR_flgHtgPwrReq/1
  BTMR_HtgFlgPwrCalc/2(BTMR_pHtgPwrReq) -> BTMR_pHtgPwrReq/1
  stBrsSts/1 -> BTMR_BrushFlgCalc/1(stBrsSts)
  stHtgSts/1 -> BTMR_HtgFlgPwrCalc/1(stHtgSts)
  stCoolSts/1 -> BTMR_CoolFlgPwrCalc/2(stCoolSts)
  BTMR_flgHtgTempSgns/1 -> BTMR_HtgFlgPwrCalc/2(BTMR_flgHtgTempSgns)
  BTMR_pHtgDCPwrSgns/1 -> BTMR_HtgFlgPwrCalc/3(BTMR_pHtgDCPwrSgns)
  BTMR_flgCoolTempSgns/1 -> BTMR_CoolFlgPwrCalc/3(BTMR_flgCoolTempSgns)
  BCMR_pHeatPwrReq/1 -> BTMR_HtgFlgPwrCalc/4(BCMR_pHeatPwrReq)
  BCMR_stAChrgPreThmReq/1 -> BTMR_HtgFlgPwrCalc/5(BCMR_stAChrgPreThmReq)
  BCMR_stHoldTempReq/1 -> BTMR_HtgFlgPwrCalc/6(BCMR_stHoldTempReq)

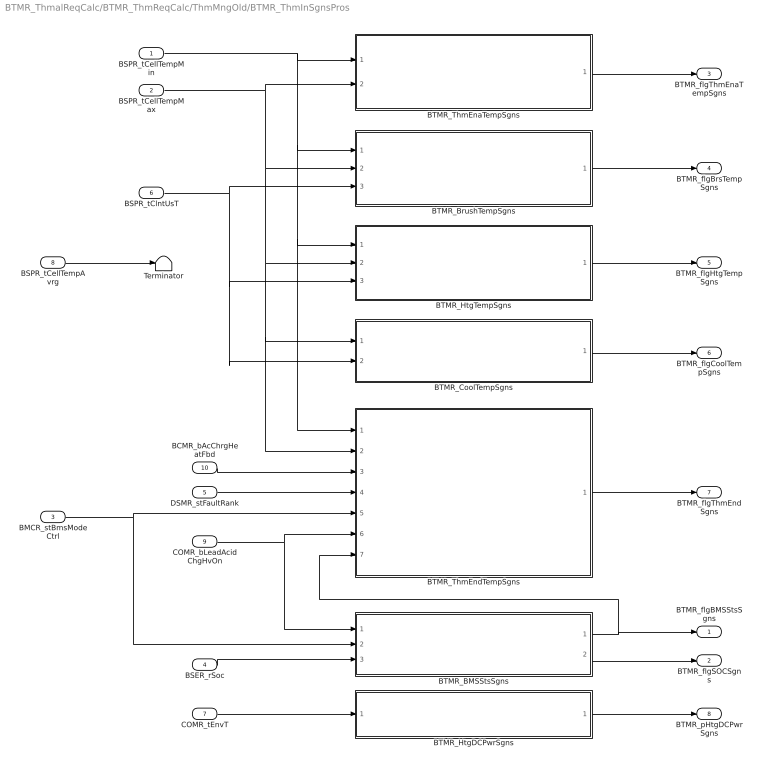
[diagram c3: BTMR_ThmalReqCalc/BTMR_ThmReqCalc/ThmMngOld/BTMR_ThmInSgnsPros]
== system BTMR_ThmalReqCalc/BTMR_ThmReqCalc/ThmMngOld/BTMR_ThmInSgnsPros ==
  BSPR_tCellTempMin : Inport
  BSPR_tCellTempMax : Inport  Port=2
  BMCR_stBmsModeCtrl : Inport  Port=3
  BSER_rSoc : Inport  Port=4
  DSMR_stFaultRank : Inport  Port=5
  BSPR_tClntUsT : Inport  Port=6
  COMR_tEnvT : Inport  Port=7
  BSPR_tCellTempAvrg : Inport  Port=8
  COMR_bLeadAcidChgHvOn : Inport  Port=9
  BCMR_bAcChrgHeatFbd : Inport  Port=10
  BTMR_BMSStsSgns : Subsystem
  BTMR_BrushTempSgns : Subsystem
  BTMR_CoolTempSgns : Subsystem
  BTMR_HtgDCPwrSgns : Subsystem
  BTMR_HtgTempSgns : Subsystem
  BTMR_ThmEnaTempSgns : Subsystem
  BTMR_ThmEndTempSgns : Subsystem
  Terminator : Terminator
  BTMR_flgBMSStsSgns : Outport
  BTMR_flgSOCSgns : Outport  Port=2
  BTMR_flgThmEnaTempSgns : Outport  Port=3
  BTMR_flgBrsTempSgns : Outport  Port=4
  BTMR_flgHtgTempSgns : Outport  Port=5
  BTMR_flgCoolTempSgns : Outport  Port=6
  BTMR_flgThmEndSgns : Outport  Port=7
  BTMR_pHtgDCPwrSgns : Outport  Port=8
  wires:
  BTMR_ThmEnaTempSgns/1(BTMR_flgThmEnaTempSgns) -> BTMR_flgThmEnaTempSgns/1
  BSPR_tClntUsT/1 -> BTMR_CoolTempSgns/2(BSPR_tClntUsT), BTMR_HtgTempSgns/3(BSPR_tClntUsT), BTMR_BrushTempSgns/3(BSPR_tClntUsT)
  BTMR_CoolTempSgns/1(BTMR_flgCoolTempSgns) -> BTMR_flgCoolTempSgns/1
  BSER_rSoc/1 -> BTMR_BMSStsSgns/3(BSER_rSoc)
  BTMR_ThmEndTempSgns/1(BTMR_flgThmEndSgns) -> BTMR_flgThmEndSgns/1
  BTMR_BMSStsSgns/1(BTMR_flgBMSSgns) -> BTMR_ThmEndTempSgns/7(BTMR_flgBMSSgns), BTMR_flgBMSStsSgns/1
  BTMR_HtgTempSgns/1(BTMR_flgHtgTempSgns) -> BTMR_flgHtgTempSgns/1
  BTMR_BrushTempSgns/1(BTMR_flgBrsTempSgns) -> BTMR_flgBrsTempSgns/1
  BTMR_BMSStsSgns/2(BTMR_flgSOCSgns) -> BTMR_flgSOCSgns/1
  BMCR_stBmsModeCtrl/1 -> BTMR_BMSStsSgns/2(BMCR_stBmsModeCtrl), BTMR_ThmEndTempSgns/5(BMCR_stBmsModeCtrl)
  DSMR_stFaultRank/1 -> BTMR_ThmEndTempSgns/4(DSMR_stFaultRank)
  BSPR_tCellTempMax/1 -> BTMR_ThmEndTempSgns/2(BSPR_tCellTempMax), BTMR_CoolTempSgns/1(BSPR_tCellTempMax), BTMR_HtgTempSgns/2(BSPR_tCellTempMax), BTMR_BrushTempSgns/2(BSPR_tCellTempMax), BTMR_ThmEnaTempSgns/2(BSPR_tCellTempMax)
  BSPR_tCellTempMin/1 -> BTMR_ThmEndTempSgns/1(BSPR_tCellTempMin), BTMR_HtgTempSgns/1(BSPR_tCellTempMin), BTMR_BrushTempSgns/1(BSPR_tCellTempMin), BTMR_ThmEnaTempSgns/1(BSPR_tCellTempMin)
  COMR_tEnvT/1 -> BTMR_HtgDCPwrSgns/1(COMR_tEnvT)
  BTMR_HtgDCPwrSgns/1(BTMR_pHtgDCPwrSgns) -> BTMR_pHtgDCPwrSgns/1
  BSPR_tCellTempAvrg/1 -> Terminator/1
  COMR_bLeadAcidChgHvOn/1 -> BTMR_BMSStsSgns/1(COMR_bLeadAcidChgHvOn), BTMR_ThmEndTempSgns/6(COMR_bLeadAcidChgHvOn)
  BCMR_bAcChrgHeatFbd/1 -> BTMR_ThmEndTempSgns/3(BCMR_bAcChrgHeatFbd)

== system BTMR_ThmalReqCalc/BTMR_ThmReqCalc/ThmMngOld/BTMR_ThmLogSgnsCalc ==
  BTMR_flgBMSStsSgns : Inport
  BTMR_flgSOCSgns : Inport  Port=2
  BTMR_flgThmEnaTempSgns : Inport  Port=3
  BTMR_flgBrsTempSgns : Inport  Port=4
  BTMR_flgHtgTempSgns : Inport  Port=5
  BTMR_flgCoolTempSgns : Inport  Port=6
  BTMR_BThmDnaLogCalc : Subsystem
  BTMR_BThmEnaLogCalc : Subsystem
  BTMR_ThmLogPreCalc : Subsystem
  BTMR_flgBTMREnaSgns : Outport
  BTMR_flgBTMRDnaSgns : Outport  Port=2
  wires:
  BTMR_flgBrsTempSgns/1 -> BTMR_BThmDnaLogCalc/2(BTMR_flgBrsTempSgns), BTMR_ThmLogPreCalc/4(BTMR_flgBrsTempSgns)
  BTMR_flgHtgTempSgns/1 -> BTMR_BThmDnaLogCalc/3(BTMR_flgHtgTempSgns)
  BTMR_flgCoolTempSgns/1 -> BTMR_BThmDnaLogCalc/4(BTMR_flgCoolTempSgns)
  BTMR_BThmDnaLogCalc/1(BTMR_flgBThmDnaSgns) -> BTMR_flgBTMRDnaSgns/1
  BTMR_flgBMSStsSgns/1 -> BTMR_ThmLogPreCalc/1(BTMR_flgBMSStsSgns)
  BTMR_flgSOCSgns/1 -> BTMR_BThmEnaLogCalc/4(BTMR_flgSOCSgns), BTMR_BThmDnaLogCalc/1(BTMR_flgSOCSgns), BTMR_ThmLogPreCalc/2(BTMR_flgSOCSgns)
  BTMR_BThmEnaLogCalc/1(BTMR_flgBTMREnaSgns) -> BTMR_flgBTMREnaSgns/1
  BTMR_ThmLogPreCalc/2(BTMR_flgHtgLogSgns) -> BTMR_BThmEnaLogCalc/2(BTMR_flgHtgLogSgns)
  BTMR_ThmLogPreCalc/1(BTMR_flgBrsLogSgns) -> BTMR_BThmEnaLogCalc/1(BTMR_flgBrsLogSgns)
  BTMR_ThmLogPreCalc/3(BTMR_flgCoolLogSgns) -> BTMR_BThmEnaLogCalc/3(BTMR_flgCoolLogSgns)
  BTMR_flgThmEnaTempSgns/1 -> BTMR_ThmLogPreCalc/3(BTMR_flgThmEnaTempSgns)

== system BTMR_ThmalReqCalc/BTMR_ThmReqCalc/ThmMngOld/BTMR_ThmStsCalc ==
  BTMR_flgBTMREnaSgns : Inport
  BTMR_flgBTMRDnaSgns : Inport  Port=2
  BTMR_flgThmEndSgns : Inport  Port=3
  BTMR_flgBrsTempSgns : Inport  Port=4
  BTMR_ThmStsCalc : Stateflow chart  TreatAsAtomicUnit=on
  Bus Selector : BusSelector  OutputSignals=BTMR_flgBrsEna,BTMR_flgHtgDCEna,BTMR_flgHtgACEna,BTMR_flgHtgDrvSEna,BTMR_flgCoolNormEna,BTMR_flgCoolChrgEna
  Bus Selector1 : BusSelector  OutputSignals=BTMR_flgBrsDna,BTMR_flgHtgDCDna,BTMR_flgHtgACDna,BTMR_flgHtgDrvDna,BTMR_flgCoolNormDna,BTMR_flgCoolChrgDna
  Bus Selector2 : BusSelector  OutputSignals=BTMR_flgBrsThmEnd,BTMR_flgHtgDCThmEnd,BTMR_flgHtgACThmEnd,BTMR_flgHtgDrvThmEnd,BTMR_flgCoolNormThmEnd,BTMR_flgCoolChrgThmEnd
  Bus Selector3 : BusSelector  OutputSignals=BTMR_flgBrsInTempSgns
  Bus Selector4 : BusSelector  OutputSignals=BTMR_flgBrsStartTemp
  Data Type Conversion : DataTypeConversion  OutDataTypeStr=uint8
  Data Type Conversion1 : DataTypeConversion  OutDataTypeStr=uint8
  Data Type Conversion2 : DataTypeConversion  OutDataTypeStr=uint8
  stBrsSts : Outport
  stHtgSts : Outport  Port=2
  stCoolSts : Outport  Port=3
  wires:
  BTMR_ThmStsCalc/2(stHtgSts) -> Data Type Conversion1/1
  BTMR_ThmStsCalc/1(stBrsSts) -> Data Type Conversion/1
  BTMR_ThmStsCalc/3(stCoolSts) -> Data Type Conversion2/1
  BTMR_flgBTMREnaSgns/1 -> Bus Selector/1
  Bus Selector/2 -> BTMR_ThmStsCalc/2(HtgDCEna)  "<BTMR_flgHtgDCEna>"
  Bus Selector/1 -> BTMR_ThmStsCalc/1(BrsEna)  "<BTMR_flgBrsEna>"
  Bus Selector/3 -> BTMR_ThmStsCalc/3(HtgACEna)  "<BTMR_flgHtgACEna>"
  Bus Selector/4 -> BTMR_ThmStsCalc/4(HtgDrvEna)  "<BTMR_flgHtgDrvSEna>"
  Bus Selector/5 -> BTMR_ThmStsCalc/5(CoolNormEna)  "<BTMR_flgCoolNormEna>"
  Bus Selector/6 -> BTMR_ThmStsCalc/6(CoolChrgEna)  "<BTMR_flgCoolChrgEna>"
  BTMR_flgBTMRDnaSgns/1 -> Bus Selector1/1
  Bus Selector1/1 -> BTMR_ThmStsCalc/7(BrsDna)  "<BTMR_flgBrsDna>"
  Bus Selector1/2 -> BTMR_ThmStsCalc/8(HtgDCDna)  "<BTMR_flgHtgDCDna>"
  Bus Selector1/3 -> BTMR_ThmStsCalc/9(HtgACDna)  "<BTMR_flgHtgACDna>"
  Bus Selector1/4 -> BTMR_ThmStsCalc/10(HtgDrvDna)  "<BTMR_flgHtgDrvDna>"
  Bus Selector1/5 -> BTMR_ThmStsCalc/11(CoolNormDna)  "<BTMR_flgCoolNormDna>"
  Bus Selector1/6 -> BTMR_ThmStsCalc/12(CoolChrgDna)  "<BTMR_flgCoolChrgDna>"
  BTMR_flgThmEndSgns/1 -> Bus Selector2/1
  Bus Selector2/2 -> BTMR_ThmStsCalc/14(HtgDCThmEnd)  "<BTMR_flgHtgDCThmEnd>"
  Bus Selector2/3 -> BTMR_ThmStsCalc/15(HtgACThmEnd)  "<BTMR_flgHtgACThmEnd>"
  Bus Selector2/4 -> BTMR_ThmStsCalc/16(HtgDrvThmEnd)  "<BTMR_flgHtgDrvThmEnd>"
  Bus Selector2/5 -> BTMR_ThmStsCalc/17(CoolNormThmEnd)  "<BTMR_flgCoolNormThmEnd>"
  Bus Selector2/6 -> BTMR_ThmStsCalc/18(CoolChrgThmEnd)  "<BTMR_flgCoolChrgThmEnd>"
  BTMR_flgBrsTempSgns/1 -> Bus Selector3/1
  Bus Selector3/1 -> Bus Selector4/1  "<BTMR_flgBrsInTempSgns>"
  Bus Selector4/1 -> BTMR_ThmStsCalc/19(BrsStart)  "<BTMR_flgBrsStartTemp>"
  Bus Selector2/1 -> BTMR_ThmStsCalc/13(BrsThmEnd)  "<BTMR_flgBrsThmEnd>"
  Data Type Conversion/1 -> stBrsSts/1
  Data Type Conversion1/1 -> stHtgSts/1
  Data Type Conversion2/1 -> stCoolSts/1

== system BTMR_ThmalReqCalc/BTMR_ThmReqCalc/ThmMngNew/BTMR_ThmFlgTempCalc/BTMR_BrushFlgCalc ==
  stBrsSts : Inport
  Constant : Constant  Value=10  OutDataTypeStr=single
  Constant1 : Constant  Value=enmThmBrsFlg.INACTIVE  OutDataTypeStr=Enum: enmThmBrsFlg
  Constant2 : Constant  Value=BMS_cntThmStbNum_C
  Constant21 : Constant  Value=enmThmBrsSts.ACTIVE  OutDataTypeStr=Enum: enmThmBrsSts
  Constant3 : Constant  Value=enmThmBrsFlg.ACTIVE  OutDataTypeStr=Enum: enmThmBrsFlg
  Constant4 : Constant  Value=BTMR_rFlashClbFlg_C
  Data Type Conversion{,1..2,4} (4 alike) : DataTypeConversion  OutDataTypeStr=uint8
  Relational Operator : RelationalOperator  Operator=>  OutDataTypeStr=boolean  RndMeth=Simplest
  Relational Operator7 : RelationalOperator  Operator===  OutDataTypeStr=boolean  RndMeth=Simplest
  Stable_Calc1 : Subsystem
  Switch1 : Switch  Criteria=u2 ~= 0
  Switch2 : Switch  Criteria=u2 ~= 0
  BTMR_flgBrsTempReq : Outport
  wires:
  Data Type Conversion2/1 -> Switch1/3
  stBrsSts/1 -> Relational Operator7/1
  Data Type Conversion1/1 -> Switch1/1
  Relational Operator7/1 -> Stable_Calc1/1(source_Uint)
  Constant21/1 -> Data Type Conversion/1
  Data Type Conversion/1 -> Relational Operator7/2
  Constant3/1 -> Data Type Conversion1/1
  Constant1/1 -> Data Type Conversion2/1
  Constant2/1 -> Stable_Calc1/2(cntStable)
  Stable_Calc1/1(stableOut) -> Switch1/2
  Constant/1 -> Relational Operator/2
  Constant4/1 -> Relational Operator/1
  Relational Operator/1 -> Data Type Conversion4/1, Switch2/2
  Switch1/1 -> Switch2/3
  Switch2/1 -> BTMR_flgBrsTempReq/1
  Data Type Conversion4/1 -> Switch2/1

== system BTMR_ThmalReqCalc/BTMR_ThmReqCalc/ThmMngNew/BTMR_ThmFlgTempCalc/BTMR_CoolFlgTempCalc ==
  BTMR_flgBrsTempReq : Inport
  stCoolSts : Inport  Port=2
  BTMR_flgCoolTempSgns : Inport  Port=3
  BTMR_CoolChrgFlgTempCalc : Subsystem
  BTMR_CoolNormFlgTempCalc : Subsystem
  BTMR_flgTemp_Out : Subsystem
  Bus Selector1 : BusSelector  OutputSignals=BTMR_flgCoolNormTempSgns,BTMR_flgCoolChrgTempSgns
  Constant1 : Constant  Value=enmThmCoolSts.CoolNorm  OutDataTypeStr=Enum: enmThmCoolSts
  Constant2 : Constant  Value=enmThmCoolSts.CoolChrg  OutDataTypeStr=Enum: enmThmCoolSts
  Data Type Conversion : DataTypeConversion  OutDataTypeStr=uint8
  Data Type Conversion1 : DataTypeConversion  OutDataTypeStr=uint8
  Merge : Merge
  Merge1 : Merge
  Relational Operator2 : RelationalOperator  Operator===  OutDataTypeStr=boolean  RndMeth=Simplest
  Relational Operator3 : RelationalOperator  Operator===  OutDataTypeStr=boolean  RndMeth=Simplest
  BTMR_flgClntTempReq : Outport
  BTMR_tClntTempReq : Outport  Port=2
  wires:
  Relational Operator3/1 -> BTMR_CoolChrgFlgTempCalc/Enable
  stCoolSts/1 -> [stCoolSts], Relational Operator3/1, Relational Operator2/1
  Data Type Conversion1/1 -> Relational Operator3/2
  Relational Operator2/1 -> BTMR_CoolNormFlgTempCalc/Enable
  Data Type Conversion/1 -> Relational Operator2/2
  BTMR_flgCoolTempSgns/1 -> Bus Selector1/1
  Bus Selector1/1 -> BTMR_CoolNormFlgTempCalc/1(BTMR_flgCoolNormTempSgns)  "<BTMR_flgCoolNormTempSgns>"
  Bus Selector1/2 -> BTMR_CoolChrgFlgTempCalc/1(BTMR_flgCoolChrgTempSgns)  "<BTMR_flgCoolChrgTempSgns>"
  Constant1/1 -> Data Type Conversion/1
  Constant2/1 -> Data Type Conversion1/1
  BTMR_CoolNormFlgTempCalc/1(BTMR_flgClntTempReq) -> Merge/1
  BTMR_CoolChrgFlgTempCalc/1(BTMR_flgClntTempReq) -> Merge/2
  BTMR_CoolChrgFlgTempCalc/2(BTMR_tClntTempReq) -> Merge1/2
  BTMR_CoolNormFlgTempCalc/2(BTMR_tClntTempReq) -> Merge1/1
  Merge/1 -> BTMR_flgTemp_Out/3(BTMR_flgClntTempReqMerge)
  BTMR_flgBrsTempReq/1 -> BTMR_flgTemp_Out/2(BTMR_flgBrsTempReq)
  [stCoolSts] -> BTMR_flgTemp_Out/1(stCoolSts)
  Merge1/1 -> BTMR_flgTemp_Out/4(BTMR_tClntTempReqMerge)
  BTMR_flgTemp_Out/1(BTMR_flgClntTempReq) -> BTMR_flgClntTempReq/1
  BTMR_flgTemp_Out/2(BTMR_tClntTempReq) -> BTMR_tClntTempReq/1

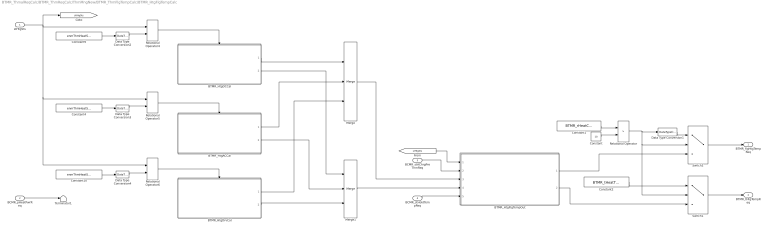
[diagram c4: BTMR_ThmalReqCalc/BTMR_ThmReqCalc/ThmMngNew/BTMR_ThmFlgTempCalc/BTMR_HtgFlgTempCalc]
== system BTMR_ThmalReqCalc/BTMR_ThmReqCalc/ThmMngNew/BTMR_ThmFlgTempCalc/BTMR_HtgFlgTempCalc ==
  stHtgSts : Inport
  BCMR_pHeatPwrReq : Inport  Port=2
  BCMR_stAChrgPreThmReq : Inport  Port=3
  BCMR_stHoldTempReq : Inport  Port=4
  BTMR_HtgACCal : Subsystem
  BTMR_HtgDCCal : Subsystem
  BTMR_HtgDrvCal : Subsystem
  BTMR_HtgFlgTempOut : Subsystem
  Constant : Constant  Value=10  OutDataTypeStr=single
  Constant1 : Constant  Value=BTMR_rHeatClbFlg_C
  Constant10 : Constant  Value=enmThmHeatSts.HeatDrv  OutDataTypeStr=Enum: enmThmHeatSts
  Constant2 : Constant  Value=BTMR_tHeatTempClbQnt_C
  Constant4 : Constant  Value=enmThmHeatSts.HeatAC  OutDataTypeStr=Enum: enmThmHeatSts
  Constant9 : Constant  Value=enmThmHeatSts.HeatDC  OutDataTypeStr=Enum: enmThmHeatSts
  Data Type Conversion{1..4} (4 alike) : DataTypeConversion  OutDataTypeStr=uint8
  Merge : Merge  Inputs=3
  Merge1 : Merge  Inputs=3
  Relational Operator : RelationalOperator  Operator=>  OutDataTypeStr=boolean  RndMeth=Simplest
  Relational Operator4 : RelationalOperator  Operator===  OutDataTypeStr=boolean  RndMeth=Simplest
  Relational Operator5 : RelationalOperator  Operator===  OutDataTypeStr=boolean  RndMeth=Simplest
  Relational Operator6 : RelationalOperator  Operator===  OutDataTypeStr=boolean  RndMeth=Simplest
  Switch1 : Switch  Criteria=u2 ~= 0
  Switch2 : Switch  Criteria=u2 ~= 0
  Terminator1 : Terminator
  BTMR_flgHtgTempReq : Outport
  BTMR_tHtgTempReq : Outport  Port=2
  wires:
  stHtgSts/1 -> [stHtgSts], Relational Operator6/1, Relational Operator5/1, Relational Operator4/1
  Relational Operator6/1 -> BTMR_HtgDrvCal/Enable
  Relational Operator4/1 -> BTMR_HtgDCCal/Enable
  BCMR_pHeatPwrReq/1 -> Terminator1/1
  Data Type Conversion2/1 -> Relational Operator4/2
  Constant9/1 -> Data Type Conversion2/1
  Data Type Conversion3/1 -> Relational Operator5/2
  Constant4/1 -> Data Type Conversion3/1
  Data Type Conversion4/1 -> Relational Operator6/2
  Constant10/1 -> Data Type Conversion4/1
  Relational Operator5/1 -> BTMR_HtgACCal/Enable
  BTMR_HtgDCCal/1(BTMR_flgHtgTempReq) -> Merge/1
  BTMR_HtgACCal/1(BTMR_flgHtgTempReq) -> Merge/2
  BTMR_HtgDrvCal/1(BTMR_flgHtgTempReq) -> Merge/3
  BTMR_HtgACCal/2(BTMR_tHtgTempReq) -> Merge1/2
  BTMR_HtgDCCal/2(BTMR_tHtgTempReq) -> Merge1/1
  BTMR_HtgDrvCal/2(BTMR_tHtgTempReq) -> Merge1/3
  Merge/1 -> BTMR_HtgFlgTempOut/3(BTMR_flgHtgTempReqMerge)
  [stHtgSts] -> BTMR_HtgFlgTempOut/1(stHtgSts)
  BCMR_stAChrgPreThmReq/1 -> BTMR_HtgFlgTempOut/2(BCMR_stAChrgPreThmReq)
  Merge1/1 -> BTMR_HtgFlgTempOut/4(BTMR_tHtgTempReqMerge)
  Constant/1 -> Relational Operator/2
  Constant1/1 -> Relational Operator/1
  Relational Operator/1 -> Data Type Conversion1/1, Switch2/2, Switch1/2
  Constant2/1 -> Switch1/1
  Switch1/1 -> BTMR_tHtgTempReq/1
  BTMR_HtgFlgTempOut/2(BTMR_tHtgTempReq) -> Switch1/3
  BTMR_HtgFlgTempOut/1(BTMR_flgHtgTempReq) -> Switch2/3
  Switch2/1 -> BTMR_flgHtgTempReq/1
  Data Type Conversion1/1 -> Switch2/1
  BCMR_stHoldTempReq/1 -> BTMR_HtgFlgTempOut/5(BCMR_stHoldTempReq)

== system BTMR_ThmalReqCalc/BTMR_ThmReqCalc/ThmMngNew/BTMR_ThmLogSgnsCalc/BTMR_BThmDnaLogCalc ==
  BTMR_flgSOCSgns : Inport
  BTMR_flgBrsTempSgns : Inport  Port=2
  BTMR_flgHtgTempSgns : Inport  Port=3
  BTMR_flgCoolTempSgns : Inport  Port=4
  BTMR_BrsDnaCalc : Subsystem
  BTMR_CoolDnaCalc : Subsystem
  BTMR_HtgDnaCalc : Subsystem
  Bus Creator : BusCreator  Inputs=6
  BTMR_flgBThmDnaSgns : Outport
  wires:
  BTMR_CoolDnaCalc/2(BTMR_flgCoolChrgDna) -> Bus Creator/6  "BTMR_flgCoolChrgDna"
  BTMR_CoolDnaCalc/1(BTMR_flgCoolNormDna) -> Bus Creator/5  "BTMR_flgCoolNormDna"
  BTMR_HtgDnaCalc/3(BTMR_flgHtgDrvDna) -> Bus Creator/4  "BTMR_flgHtgDrvDna"
  BTMR_HtgDnaCalc/2(BTMR_flgHtgACDna) -> Bus Creator/3  "BTMR_flgHtgACDna"
  BTMR_HtgDnaCalc/1(BTMR_flgHtgDCDna) -> Bus Creator/2  "BTMR_flgHtgDCDna"
  BTMR_flgCoolTempSgns/1 -> BTMR_CoolDnaCalc/1(BTMR_flgCoolLogSgns)
  BTMR_flgHtgTempSgns/1 -> BTMR_HtgDnaCalc/1(BTMR_flgHtgLogSgns)
  BTMR_BrsDnaCalc/1(BTMR_flgBrsDna) -> Bus Creator/1  "BTMR_flgBrsDna"
  Bus Creator/1 -> BTMR_flgBThmDnaSgns/1  "BTMR_flgBThmDnaSgns"
  BTMR_flgBrsTempSgns/1 -> BTMR_BrsDnaCalc/1(BTMR_flgBrsLogSgns)
  BTMR_flgSOCSgns/1 -> BTMR_HtgDnaCalc/2(BTMR_flgSOCSgns)

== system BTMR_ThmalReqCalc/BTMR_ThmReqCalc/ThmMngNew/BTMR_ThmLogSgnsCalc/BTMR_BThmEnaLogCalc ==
  BTMR_flgBrsLogSgns : Inport
  BTMR_flgHtgLogSgns : Inport  Port=2
  BTMR_flgCoolLogSgns : Inport  Port=3
  BTMR_flgSOCSgns : Inport  Port=4
  BTMR_BrsEnaCalc : Subsystem
  BTMR_CoolEnaCalc : Subsystem
  BTMR_HtgEnaCalc : Subsystem
  Bus Creator : BusCreator  Inputs=6
  BTMR_flgBTMREnaSgns : Outport
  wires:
  BTMR_flgBrsLogSgns/1 -> BTMR_BrsEnaCalc/1(BTMR_flgBrsLogSgns)
  Bus Creator/1 -> BTMR_flgBTMREnaSgns/1  "BTMR_flgBTMREnaSgns"
  BTMR_BrsEnaCalc/1(BTMR_flgBrsEna) -> Bus Creator/1
  BTMR_flgHtgLogSgns/1 -> BTMR_HtgEnaCalc/1(BTMR_flgHtgLogSgns)
  BTMR_flgCoolLogSgns/1 -> BTMR_CoolEnaCalc/1(BTMR_flgCoolLogSgns)
  BTMR_HtgEnaCalc/1(BTMR_flgHtgDCEna) -> Bus Creator/2
  BTMR_HtgEnaCalc/2(BTMR_flgHtgACEna) -> Bus Creator/3
  BTMR_HtgEnaCalc/3(BTMR_flgHtgDrvEna) -> Bus Creator/4
  BTMR_CoolEnaCalc/1(BTMR_flgCoolNormEna) -> Bus Creator/5
  BTMR_CoolEnaCalc/2(BTMR_flgCoolChrgEna) -> Bus Creator/6
  BTMR_flgSOCSgns/1 -> BTMR_HtgEnaCalc/2(BTMR_flgSOCSgns)

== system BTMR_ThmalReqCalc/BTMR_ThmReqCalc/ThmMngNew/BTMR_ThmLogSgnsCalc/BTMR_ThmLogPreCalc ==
  BTMR_flgBMSStsSgns : Inport
  BTMR_flgSOCSgns : Inport  Port=2
  BTMR_flgThmEnaTempSgns : Inport  Port=3
  BTMR_flgBrsTempSgns : Inport  Port=4
  BTMR_BrsLogCalc : Subsystem
  BTMR_CoolLogCalc : Subsystem
  BTMR_HtgLogCalc : Subsystem
  BTMR_flgBrsLogSgns : Outport
  BTMR_flgHtgLogSgns : Outport  Port=2
  BTMR_flgCoolLogSgns : Outport  Port=3
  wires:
  BTMR_flgBMSStsSgns/1 -> BTMR_BrsLogCalc/1(BTMR_flgBMSStsSgns)
  BTMR_flgBrsTempSgns/1 -> BTMR_BrsLogCalc/3(BTMR_flgBrsTempSgns)
  BTMR_flgSOCSgns/1 -> BTMR_BrsLogCalc/2(BTMR_flgSOCSgns)
  BTMR_BrsLogCalc/1(BTMR_flgBrsLogSgns) -> BTMR_HtgLogCalc/1(BTMR_flgBrsLogSgns), BTMR_flgBrsLogSgns/1
  BTMR_CoolLogCalc/1(BTMR_flgCoolLogSgns) -> BTMR_flgCoolLogSgns/1
  BTMR_HtgLogCalc/1(BTMR_flgHtgLogSgns) -> BTMR_flgHtgLogSgns/1, BTMR_CoolLogCalc/1(BTMR_flgHtgLogSgns)
  BTMR_flgThmEnaTempSgns/1 -> BTMR_CoolLogCalc/2(BTMR_flgThmEnaTempSgns), BTMR_HtgLogCalc/2(BTMR_flgThmEnaTempSgns)

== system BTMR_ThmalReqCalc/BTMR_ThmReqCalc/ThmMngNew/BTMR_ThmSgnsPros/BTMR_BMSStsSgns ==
  COMR_bLeadAcidChgHvOn : Inport
  BMCR_stBmsModeCtrl : Inport  Port=2
  BSER_rSoc : Inport  Port=3
  BTMR_BmsStsCalc : Subsystem
  BTMR_SOCStsCalc : Subsystem
  BTMR_flgBMSSgns : Outport
  BTMR_flgSOCSgns : Outport  Port=2
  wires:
  BSER_rSoc/1 -> BTMR_SOCStsCalc/1(BSER_rSoc)
  BMCR_stBmsModeCtrl/1 -> BTMR_BmsStsCalc/1(BMCR_stBmsModeCtrl)
  BTMR_SOCStsCalc/1(BTMR_flgSOCSgns) -> BTMR_flgSOCSgns/1
  BTMR_BmsStsCalc/1(BTMR_flgBMSSgns) -> BTMR_flgBMSSgns/1
  COMR_bLeadAcidChgHvOn/1 -> BTMR_BmsStsCalc/2(COMR_bLeadAcidChgHvOn)

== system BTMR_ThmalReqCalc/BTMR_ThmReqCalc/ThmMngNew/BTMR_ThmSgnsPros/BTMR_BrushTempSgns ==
  BSPR_tCellTempMin : Inport
  BSPR_tCellTempMax : Inport  Port=2
  BSPR_tClntUsT : Inport  Port=3
  BTMR_BrsCellClntTempCalc : Subsystem
  BTMR_BrsDnaTempCalc : Subsystem
  BTMR_BrsEna1TempCalc : Subsystem
  BTMR_BrsEna2TempCalc : Subsystem
  BTMR_BrsEna3TempCalc : Subsystem
  BTMR_BrsIntEna1TempCalc : Subsystem
  BTMR_BrsIntEna2TempCalc : Subsystem
  BTMR_BrsIntEna3TempCalc : Subsystem
  BTMR_BrsStartTempCalc : Subsystem
  Bus Creator : BusCreator  Inputs=2
  Bus Creator1 : BusCreator  Inputs=3
  Bus Creator2 : BusCreator  Inputs=3
  Bus Creator3 : BusCreator  Inputs=4
  BTMR_flgBrsTempSgns : Outport
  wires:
  BTMR_BrsEna2TempCalc/1(BTMR_flgBrsEna2Temp) -> Bus Creator1/2  "BTMR_flgBrsEna2Temp"
  BTMR_BrsEna1TempCalc/1(BTMR_flgBrsEna1Temp) -> Bus Creator1/1  "BTMR_flgBrsEna1Temp"
  BTMR_BrsStartTempCalc/1(BTMR_flgBrsStartTemp) -> Bus Creator/1  "BTMR_flgBrsStartTemp"
  BSPR_tCellTempMin/1 -> BTMR_BrsCellClntTempCalc/3(BSPR_tCellTempMin), BTMR_BrsEna3TempCalc/1(BSPR_tCellTempMin), BTMR_BrsEna2TempCalc/1(BSPR_tCellTempMin), BTMR_BrsEna1TempCalc/1(BSPR_tCellTempMin), BTMR_BrsDnaTempCalc/1(BSPR_tCellTempMin), BTMR_BrsStartTempCalc/1(BSPR_tCellTempMin)
  BSPR_tCellTempMax/1 -> BTMR_BrsCellClntTempCalc/1(BSPR_tCellTempMax), BTMR_BrsEna3TempCalc/2(BSPR_tCellTempMax), BTMR_BrsEna2TempCalc/2(BSPR_tCellTempMax), BTMR_BrsEna1TempCalc/2(BSPR_tCellTempMax), BTMR_BrsDnaTempCalc/2(BSPR_tCellTempMax), BTMR_BrsStartTempCalc/2(BSPR_tCellTempMax)
  BSPR_tClntUsT/1 -> BTMR_BrsCellClntTempCalc/2(BSPR_tClntUsT), BTMR_BrsIntEna3TempCalc/1(BSPR_tClntUsT), BTMR_BrsIntEna1TempCalc/1(BSPR_tClntUsT), BTMR_BrsIntEna2TempCalc/1(BSPR_tClntUsT)
  BTMR_BrsDnaTempCalc/1(BTMR_flgBrsDnaTemp) -> Bus Creator/2  "BTMR_flgBrsDnaTemp"
  BTMR_BrsEna3TempCalc/1(BTMR_flgBrsEna3Temp) -> Bus Creator1/3  "BTMR_flgBrsEna3Temp"
  BTMR_BrsIntEna1TempCalc/1(BTMR_flgBrsIntEna1Temp) -> Bus Creator2/1  "BTMR_flgBrsIntEna1Temp"
  BTMR_BrsIntEna2TempCalc/1(BTMR_flgBrsIntEna2Temp) -> Bus Creator2/2  "BTMR_flgBrsIntEna2Temp"
  BTMR_BrsIntEna3TempCalc/1(BTMR_flgBrsIntEna3Temp) -> Bus Creator2/3  "BTMR_flgBrsIntEna3Temp"
  Bus Creator/1 -> Bus Creator3/1  "BTMR_flgBrsInTempSgns"
  Bus Creator1/1 -> Bus Creator3/2  "BTMR_flgBrsEnTempSgns"
  Bus Creator2/1 -> Bus Creator3/3  "BTMR_flgBrsIntTempSgns"
  Bus Creator3/1 -> BTMR_flgBrsTempSgns/1
  BTMR_BrsCellClntTempCalc/1(BTMR_flgBrsCellClntTemp) -> Bus Creator3/4  "BTMR_flgBrsCellIntTempSgn"

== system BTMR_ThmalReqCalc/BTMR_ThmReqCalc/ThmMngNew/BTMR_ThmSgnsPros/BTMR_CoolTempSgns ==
  BSPR_tCellTempMax : Inport
  BTMR_CoolChrgTempCalc : Subsystem
  BTMR_CoolNormTempCalc : Subsystem
  Bus Creator : BusCreator  Inputs=2
  BTMR_flgCoolTempSgns : Outport
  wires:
  BSPR_tCellTempMax/1 -> BTMR_CoolChrgTempCalc/1(BSPR_tCellTempMax), BTMR_CoolNormTempCalc/1(BSPR_tCellTempMax)
  Bus Creator/1 -> BTMR_flgCoolTempSgns/1  "BTMR_flgCoolTempSgns"
  BTMR_CoolChrgTempCalc/1(BTMR_flgCoolChrgTempSgns) -> Bus Creator/2
  BTMR_CoolNormTempCalc/1(BTMR_flgCoolNormTempSgns) -> Bus Creator/1

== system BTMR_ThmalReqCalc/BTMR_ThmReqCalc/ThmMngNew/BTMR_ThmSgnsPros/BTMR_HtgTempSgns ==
  BSPR_tCellTempMin : Inport
  BSPR_tCellTempMax : Inport  Port=2
  BTMR_HtgACTempCalc : Subsystem
  BTMR_HtgDCTempCalc : Subsystem
  BTMR_HtgDrvTempCalc : Subsystem
  Bus Creator : BusCreator  Inputs=3
  BTMR_flgHtgTempSgns : Outport
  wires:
  BSPR_tCellTempMin/1 -> BTMR_HtgDrvTempCalc/1(BSPR_tCellTempMin), BTMR_HtgACTempCalc/1(BSPR_tCellTempMin), BTMR_HtgDCTempCalc/1(BSPR_tCellTempMin)
  BSPR_tCellTempMax/1 -> BTMR_HtgDrvTempCalc/2(BSPR_tCellTempMax), BTMR_HtgACTempCalc/2(BSPR_tCellTempMax), BTMR_HtgDCTempCalc/2(BSPR_tCellTempMax)
  BTMR_HtgACTempCalc/1(BTMR_flgHtgACTempSgns) -> Bus Creator/2
  BTMR_HtgDCTempCalc/1(BTMR_flgHtgDCTempSgns) -> Bus Creator/1
  BTMR_HtgDrvTempCalc/1(BTMR_flgHtgDrvTempSgns) -> Bus Creator/3
  Bus Creator/1 -> BTMR_flgHtgTempSgns/1  "BTMR_flgHtgTempSgns"

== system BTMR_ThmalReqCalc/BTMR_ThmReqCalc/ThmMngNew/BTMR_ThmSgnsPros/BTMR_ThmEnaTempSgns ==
  BSPR_tCellTempMin : Inport
  BSPR_tCellTempMax : Inport  Port=2
  BTMR_CoolChrgEnaTempCalc : Subsystem
  BTMR_CoolNormEnaTempCalc : Subsystem
  BTMR_HtgACEnaTempCalc : Subsystem
  BTMR_HtgDCEnaTempCalc : Subsystem
  BTMR_HtgDrvEnaTempCalc : Subsystem
  Bus Creator : BusCreator  Inputs=5
  Bus Creator1 : BusCreator  Inputs=2
  Bus Selector{1..5} (5 alike) : BusSelector  OutputSignals=BSPR_tCellTempMin,BSPR_tCellTempMax
  BTMR_flgThmEnaTempSgns : Outport
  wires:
  Bus Creator/1 -> BTMR_flgThmEnaTempSgns/1
  BTMR_CoolChrgEnaTempCalc/1(BTMR_flgCoolChrgEnaTemp) -> Bus Creator/5  "BTMR_CoolChrgEnaTemp"
  BTMR_CoolNormEnaTempCalc/1(BTMR_flgCoolNormEnaTemp) -> Bus Creator/4  "BTMR_CoolNormEnaTemp"
  BTMR_HtgDrvEnaTempCalc/1(BTMR_flgHtgDrvEnaTemp) -> Bus Creator/3  "BTMR_HtgDrvEnaTemp"
  BTMR_HtgDCEnaTempCalc/1(BTMR_flgHtgDCEnaTemp) -> Bus Creator/1  "BTMR_HtgDCEnaTemp"
  BTMR_HtgACEnaTempCalc/1(BTMR_flgHtgACEnaTemp) -> Bus Creator/2  "BTMR_HtgACEnaTemp"
  BSPR_tCellTempMax/1 -> Bus Creator1/2
  BSPR_tCellTempMin/1 -> Bus Creator1/1
  Bus Creator1/1 -> Bus Selector5/1, Bus Selector4/1, Bus Selector2/1, Bus Selector1/1, Bus Selector3/1
  Bus Selector1/1 -> BTMR_HtgDCEnaTempCalc/1(BSPR_tCellTempMin)  "<BSPR_tCellTempMin>"
  Bus Selector1/2 -> BTMR_HtgDCEnaTempCalc/2(BSPR_tCellTempMax)  "<BSPR_tCellTempMax>"
  Bus Selector2/1 -> BTMR_HtgACEnaTempCalc/1(BSPR_tCellTempMin)  "<BSPR_tCellTempMin>"
  Bus Selector2/2 -> BTMR_HtgACEnaTempCalc/2(BSPR_tCellTempMax)  "<BSPR_tCellTempMax>"
  Bus Selector3/1 -> BTMR_HtgDrvEnaTempCalc/1(BSPR_tCellTempMin)  "<BSPR_tCellTempMin>"
  Bus Selector3/2 -> BTMR_HtgDrvEnaTempCalc/2(BSPR_tCellTempMax)  "<BSPR_tCellTempMax>"
  Bus Selector5/1 -> BTMR_CoolChrgEnaTempCalc/1(BSPR_tCellTempMin)  "<BSPR_tCellTempMin>"
  Bus Selector5/2 -> BTMR_CoolChrgEnaTempCalc/2(BSPR_tCellTempMax)  "<BSPR_tCellTempMax>"
  Bus Selector4/1 -> BTMR_CoolNormEnaTempCalc/1(BSPR_tCellTempMin)  "<BSPR_tCellTempMin>"
  Bus Selector4/2 -> BTMR_CoolNormEnaTempCalc/2(BSPR_tCellTempMax)  "<BSPR_tCellTempMax>"
